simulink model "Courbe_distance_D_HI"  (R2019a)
settings: Solver=VariableStepAuto  StartTime=0.0  StopTime=6.283185307  MaxStep=0.001  RelTol=1e-6  SampleTimeConstraint=STIndependent

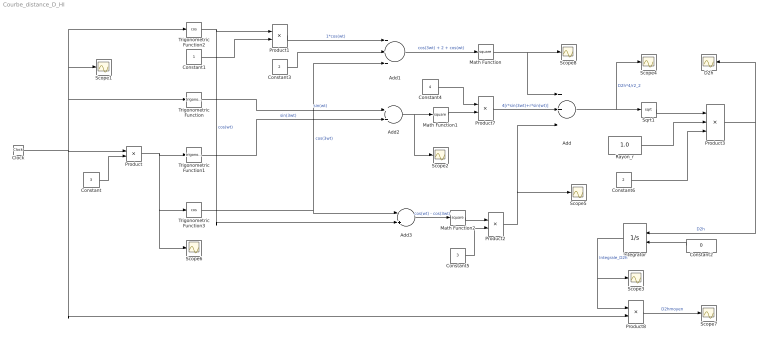
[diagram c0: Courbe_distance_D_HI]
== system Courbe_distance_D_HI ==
  Add : Sum  Inputs=+++
  Add1 : Sum  Inputs=+++
  Add2 : Sum
  Add3 : Sum  Inputs=-+
  Clock : Clock
  Constant : Constant  Value=3
  Constant1 : Constant
  Constant2 : Constant  Value=0
  Constant3 : Constant  Value=2
  Constant4 : Constant  Value=4
  Constant5 : Constant  Value=3
  Constant6 : Constant  Value=2
  D2h : Scope
  Integrator : Integrator  InitialConditionSource=external
  Math Function : Math  Operator=square
  Math Function1 : Math  Operator=square
  Math Function2 : Math  Operator=square
  Product{,1..2,7} (4 alike) : Product
  Product3 : Product  Inputs=**/
  Product8 : Product  Inputs=*/
  Rayon_r : Constant  Value=1.0
  Scope{1..8} (8 alike) : Scope
  Sqrt1 : Sqrt
  Trigonometric Function : Trigonometry
  Trigonometric Function1 : Trigonometry
  Trigonometric Function2 : Trigonometry  Operator=cos
  Trigonometric Function3 : Trigonometry  Operator=cos
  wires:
  Product/1 -> Scope6/1, Trigonometric Function3/1, Trigonometric Function1/1
  Constant/1 -> Product/2
  Clock/1 -> Product8/2, Trigonometric Function/1, Trigonometric Function2/1, Scope1/1, Product/1
  Trigonometric Function2/1 -> Add3/2, Product1/1  "cos(wt)"
  Product1/1 -> Add1/1  "1*cos(wt)"
  Add1/1 -> Math Function/1  "cos(3wt) + 2 + cos(wt)"
  Add2/1 -> Scope2/1, Math Function1/1
  Add3/1 -> Math Function2/1  "cos(wt) - cos(3wt)"
  Math Function/1 -> Scope8/1, Add/1
  Add/1 -> Sqrt1/1, Scope4/1  "D2h*4/r2_2"
  Integrator/1 -> Product8/1, Scope3/1  "Integrale_D2h"
  Constant2/1 -> Integrator/2
  Product8/1 -> Scope7/1  "D2hmoyen"
  Constant1/1 -> Product1/2
  Trigonometric Function3/1 -> Add3/1, Add1/3  "cos(3wt)"
  Constant3/1 -> Add1/2
  Trigonometric Function1/1 -> Add2/2  "sin(3wt)"
  Trigonometric Function/1 -> Add2/1  "sin(wt)"
  Math Function1/1 -> Product7/2
  Constant4/1 -> Product7/1
  Math Function2/1 -> Product2/1
  Constant5/1 -> Product2/2
  Product7/1 -> Add/2  "4[r*sin(3wt)+r*sin(wt)]"
  Product2/1 -> Add/3, Scope5/1
  Sqrt1/1 -> Product3/1
  Rayon_r/1 -> Product3/2
  Constant6/1 -> Product3/3
  Product3/1 -> Integrator/1, D2h/1  "D2h"
